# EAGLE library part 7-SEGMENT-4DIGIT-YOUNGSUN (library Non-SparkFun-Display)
This is a part for the 4-Digit 7-segment LEDs from Young Sun. Different from the Digikey LEDs, all 16 pins are used. The LONGPADS Variant is used for a test jig, but you may like it because there is more pad to solder to. If you are concerned about routing space, the standard works just fine though.
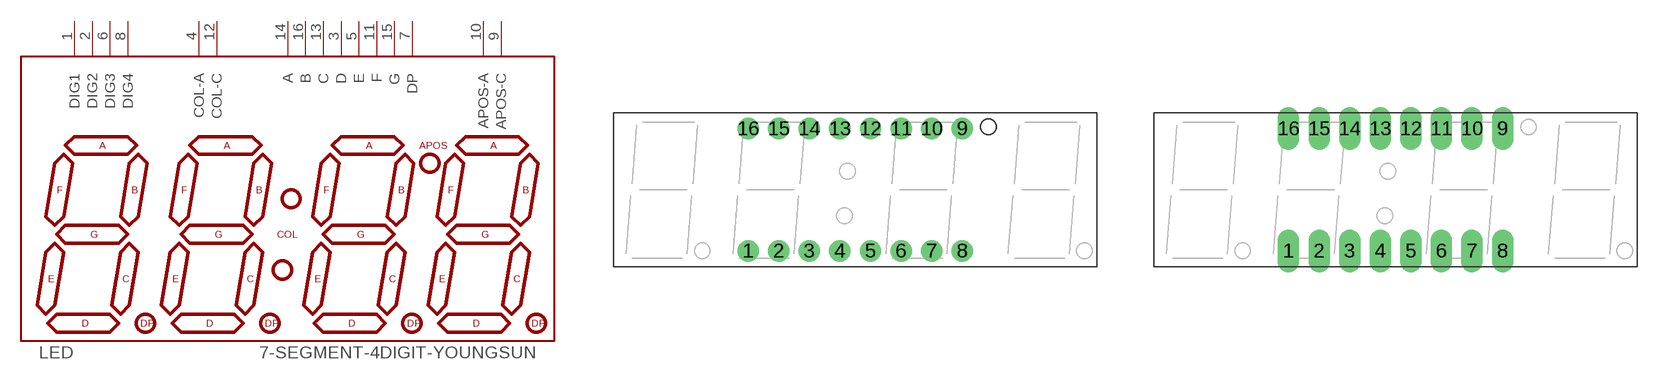
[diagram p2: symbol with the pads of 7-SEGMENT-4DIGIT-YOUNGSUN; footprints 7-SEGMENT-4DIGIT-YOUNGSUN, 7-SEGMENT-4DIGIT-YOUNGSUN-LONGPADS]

Designator prefix LED

## 7-SEGMENT-4DIGIT-YOUNGSUN  [7-SEGMENT-4DIGIT-YOUNGSUN]
1  DIG1
2  DIG2
3  D
4  COL-A
5  E
6  DIG3
7  DP
8  DIG4
9  APOS-C
10  APOS-A
11  F
12  COL-C
13  C
14  A
15  G
16  B

## 7-SEGMENT-4DIGIT-YOUNGSUNLONGPADS  [7-SEGMENT-4DIGIT-YOUNGSUN-LONGPADS]
Pads as for 7-SEGMENT-4DIGIT-YOUNGSUN

## Footprint 7-SEGMENT-4DIGIT-YOUNGSUN (pad centres in mm)
This is a package for the 4-digit 7-segment RED LED from Young Sun.
drill 0.8 pad 1.778: 1 -8.89,-5.08; 2 -6.35,-5.08; 3 -3.81,-5.08; 4 -1.27,-5.08; 5 1.27,-5.08; 6 3.81,-5.08; 7 6.35,-5.08; 8 8.89,-5.08; 9 8.89,5.08; 10 6.35,5.08; 11 3.81,5.08; 12 1.27,5.08; 13 -1.27,5.08; 14 -3.81,5.08; 15 -6.35,5.08; 16 -8.89,5.08

## Footprint 7-SEGMENT-4DIGIT-YOUNGSUN-LONGPADS (pad centres in mm)
drill 1.016 pad 1.778 long: 1 -8.89,-5.08; 2 -6.35,-5.08; 3 -3.81,-5.08; 4 -1.27,-5.08; 5 1.27,-5.08; 6 3.81,-5.08; 7 6.35,-5.08; 8 8.89,-5.08; 9 8.89,5.08; 10 6.35,5.08; 11 3.81,5.08; 12 1.27,5.08; 13 -1.27,5.08; 14 -3.81,5.08; 15 -6.35,5.08; 16 -8.89,5.08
